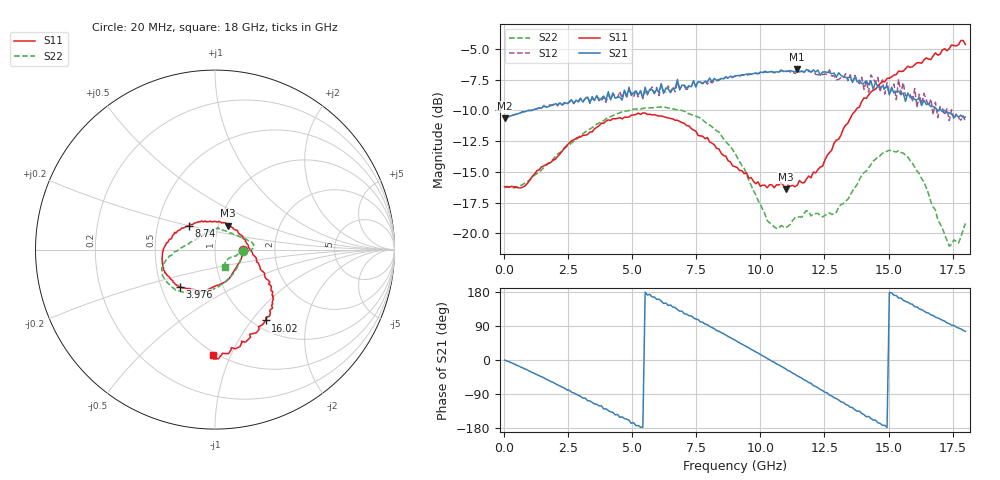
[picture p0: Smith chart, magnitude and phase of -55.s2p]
!Agilent Technologies,N5230A,US43500223,A.07.50.48
!Agilent N5230A: A.07.50.48
!Date: Sunday, January 10, 2016 19:16:13
!Correction: S11(Full 2 Port(1,2))
!S21(Full 2 Port(1,2))
!S12(Full 2 Port(1,2))
!S22(Full 2 Port(1,2))
!S2P File: Measurements: S11, S21, S12, S22:
# Hz S  dB  R 50
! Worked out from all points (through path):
!   201 points, 20 MHz to 18 GHz, reference 50 ohm
!   highest |S21| = -6.62 dB at 11.44 GHz (marker M1); lowest = -10.6 dB at 20 MHz (marker M2)
!   group delay of S21, straight-line fit = 102 ps
!   lowest |S11| = -16.4 dB at 10.99 GHz (marker M3), VSWR 1.36, Z = 55.5 + j15.1 ohm
!   |S11| at or under -10 dB: start of sweep to 13.72 GHz
!   |S22| runs from -21.0 to -9.7 dB; largest |S21 - S12| = 0.069
!   S11 on the Smith chart (normalised r, x): 20 MHz: 1.37, -0.01; 3.976 GHz: 0.62, -0.28; 8.74 GHz: 0.72, +0.20; 16.02 GHz: 1.14, -1.18; 18 GHz: 0.48, -0.86
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2e7  -16.22 -1.6  -10.63 -0.3  -10.66 -0.3  -16.26 -1.9
1.5483e9  -14.52 -71.7  -9.65 -46.9  -9.59 -47.2  -14.65 -70.2
3.0766e9  -12.01 -113.7  -9.32 -100.7  -9.23 -100.5  -11.89 -109.7
3.9756e9  -10.87 -133.4  -9.17 -128.9  -9.34 -130.1  -10.69 -125.4
5.1443e9  -10.32 -154.7  -8.40 -173.2  -8.40 -174.0  -9.88 -140.6
6.0433e9  -10.45 -167.9  -8.55 160.2  -8.79 157.5  -9.73 -151.7
7.3918e9  -11.60 169.0  -7.57 111.3  -7.66 111.3  -10.37 -164.2
8.7403e9  -14.09 137.9  -7.35 62.3  -7.37 60.9  -12.74 -175.5
9.01e9  -14.57 128.7  -7.19 52.5  -7.22 51.5  -13.49 -177.8
1.01787e10  -16.09 89.2  -6.80 8.0  -6.89 6.1  -18.44 150.6
1.09878e10  -16.43 61.8  -6.80 -23.5  -6.85 -25.6  -19.53 108.6
1.14373e10  -16.09 44.3  -6.62 -41.8  -6.87 -42.6  -18.68 92.9
1.20666e10  -15.02 18.1  -6.70 -67.3  -6.79 -67.7  -18.39 75.8
1.26959e10  -13.43 -7.8  -6.91 -92.5  -6.69 -94.0  -18.34 59.0
1.37747e10  -9.82 -29.2  -7.66 -135.3  -7.54 -138.4  -16.02 25.7
1.43141e10  -8.50 -33.3  -7.60 -154.4  -7.10 -150.6  -14.41 15.7
1.45838e10  -8.02 -36.0  -8.05 -165.6  -7.31 -169.7  -13.77 12.0
1.50333e10  -7.37 -41.0  -8.73 178.1  -8.58 175.0  -13.23 7.4
1.60222e10  -6.28 -54.5  -9.12 140.5  -8.21 137.8  -14.60 -2.2
1.61121e10  -6.12 -57.3  -9.12 140.3  -9.75 137.1  -14.94 -3.3
1.73707e10  -4.97 -80.8  -10.20 95.8  -10.83 91.4  -21.05 -35.2
1.8e10  -4.62 -91.1  -10.54 76.0  -10.92 72.9  -19.20 -60.5
